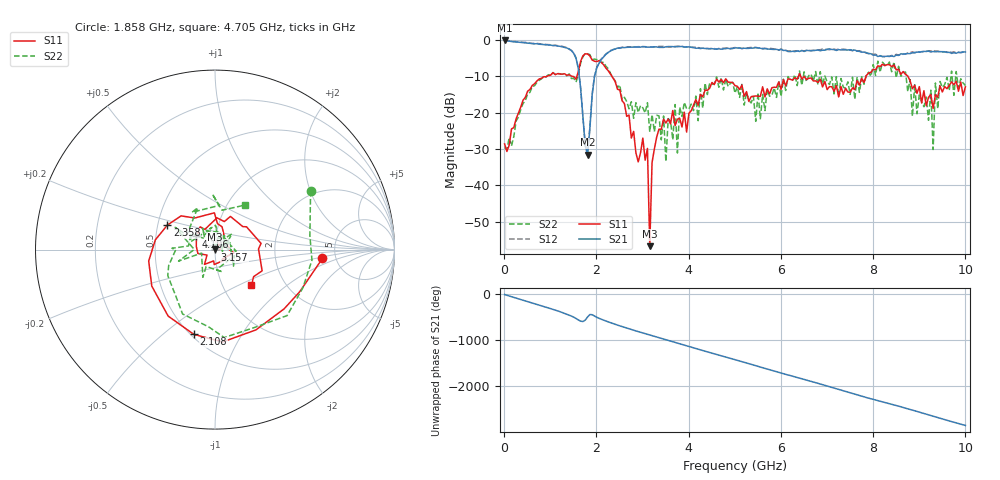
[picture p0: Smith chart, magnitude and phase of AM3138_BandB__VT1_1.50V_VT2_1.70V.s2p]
! Date/Time: Tue, Nov 13, 2018 4:39 PM
! Network Analyzer: Agilent Technologies E8364B Rev: A.07.50.67
! Sweep from 0.010 to 10.000 GHz, 201 Points, Sweep Type: LIN
! Power Supply: 1.500 V, 0.000 A
# Hz S DB R 50
!freq MagS11 AngS11 MagS21 AngS21 MagS12 AngS12 MagS22 AngS22
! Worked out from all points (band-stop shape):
!   201 points, 10 MHz to 10 GHz, reference 50 ohm
!   highest |S21| = -0.18 dB at 10 MHz (marker M1); lowest = -31.6 dB at 1.808 GHz (marker M2)
!   |S21| within 3 dB of the highest: start of sweep to 1.472 GHz; 2.292 GHz to 6.148 GHz (3.856 GHz wide, 91.4 % of centre)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
!   lowest |S11| = -56.7 dB at 3.157 GHz (marker M3), VSWR 1.00, Z = 49.9 + j0.0727 ohm
!   |S11| at or under -10 dB: 2.334 GHz to 6.381 GHz (4.047 GHz wide, 92.9 % of centre); 6.427 GHz to 7.848 GHz (1.421 GHz wide, 19.9 % of centre); 8.752 GHz to end of sweep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
!   |S22| runs from -33.5 to -3.7 dB; largest |S21 - S12| = 0.029
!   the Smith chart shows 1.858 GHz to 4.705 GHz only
!   S11 on the Smith chart (normalised r, x): 1.858 GHz: 3.91, -0.60; 2.108 GHz: 0.52, -0.64; 2.358 GHz: 0.56, +0.17; 3.157 GHz: 1.00, +0.00; 4.106 GHz: 0.80, +0.12; 4.705 GHz: 1.36, -0.59
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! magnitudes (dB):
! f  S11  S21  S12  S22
! 10 MHz  -28.6  -0.2  -0.2  -29.6
! 1.459 GHz  -10.0  -3.0  -2.9  -10.7
! 1.708 GHz  -4.4  -21.3  -21.3  -4.7
! 1.808 GHz  -3.9  -31.6  -31.4  -3.8
! 1.858 GHz  -4.4  -24.5  -24.1  -4.1
! 2.108 GHz  -6.3  -5.4  -5.2  -6.3
! 2.358 GHz  -10.5  -2.7  -2.7  -10.4
! 3.107 GHz  -29.9  -2.0  -2.0  -17.3
! 3.157 GHz  -56.7  -2.0  -2.0  -25.3
! 3.207 GHz  -33.7  -2.0  -2.0  -20.6
! 3.357 GHz  -24.6  -2.1  -1.8  -20.9
! 3.507 GHz  -22.9  -1.9  -1.9  -33.5
! 3.706 GHz  -23.6  -1.9  -1.8  -17.8
! 4.106 GHz  -17.9  -2.2  -2.0  -19.5
! 4.705 GHz  -10.9  -2.6  -2.4  -10.4
! 5.005 GHz  -12.6  -2.2  -2.1  -14.7
! 6.703 GHz  -11.3  -3.0  -2.9  -11.4
! 8.352 GHz  -6.8  -4.6  -4.5  -6.1
! 9.251 GHz  -15.0  -3.3  -3.1  -13.9
! 9.301 GHz  -18.8  -3.2  -2.9  -30.2
! 9.351 GHz  -15.1  -3.3  -3.1  -11.9
! 10 GHz  -12.9  -3.4  -3.3  -12.5
